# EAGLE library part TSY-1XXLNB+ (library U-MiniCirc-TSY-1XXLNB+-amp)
Low Power, Low Noise, MMIC Amplifier TSY-13LNB+: 0.03 - 1.0 GHz Operational Bandwidth Source: Datasheet TSY-172LNB+: 0.03 - 1.7 GHz Operational Bandwidth Source: Datasheet
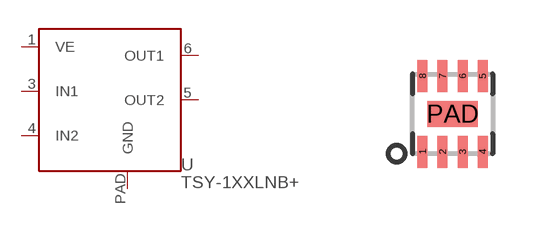
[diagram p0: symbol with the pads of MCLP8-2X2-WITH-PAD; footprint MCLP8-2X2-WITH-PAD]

Designator prefix U

## TSY-1XXLNB+  [MCLP8-2X2-WITH-PAD]
1  VE  in
3  IN1  in
4  IN2  in
5  OUT2  out
6  OUT1  out
PAD  GND  pwr

## Footprint MCLP8-2X2-WITH-PAD (pad centres in mm)
smd 0.25 x 0.8: 1 -0.75,-0.95; 2 -0.25,-0.95; 3 0.25,-0.95; 4 0.75,-0.95; 5 0.75,0.95; 6 0.25,0.95; 7 -0.25,0.95; 8 -0.75,0.95
smd 1.25 x 0.65: PAD 0,0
